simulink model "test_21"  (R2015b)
settings: Solver=FixedStepDiscrete  StartTime=0.0  StopTime=400.0  RelTol=1e-3
undefined symbols (not defined in the file or in its folder): fir1
libraries: simulink x1, dspstat3 x1

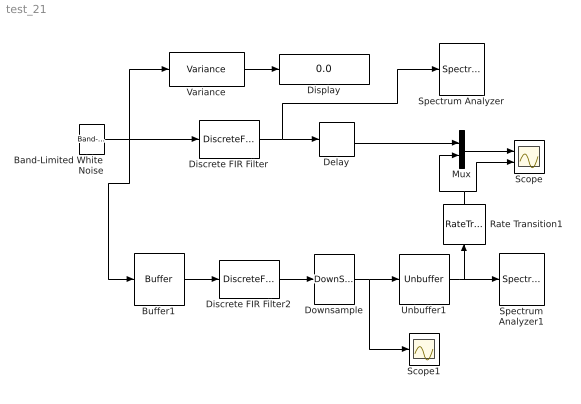
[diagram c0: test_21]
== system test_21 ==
  Band-Limited White Noise : simulink/Sources/Band-Limited White Noise  Cov=[0.01]  Ts=0.01  seed=[23341]
  Buffer1 : Buffer  N=2048  TreatMby1Signals=One channel  OutputFrames=off
  Delay : Delay  DelayLength=9*2048+4
  Discrete FIR Filter : DiscreteFir  Coefficients=fir1(256, 0.2);
  Discrete FIR Filter2 : DiscreteFir  Coefficients=fir1(256, 0.2);  InputProcessing=Columns as channels (frame based)
  Display : Display
  Downsample : DownSample  N=4  RateOptions=Allow multirate processing
  Mux : Mux  Inputs=2
  Rate Transition1 : RateTransition
  Scope : Scope  NumInputPorts=2
  Scope1 : Scope
  Spectrum Analyzer : SpectrumAnalyzer
  Spectrum Analyzer1 : SpectrumAnalyzer
  Unbuffer1 : Unbuffer  SampleBasedProcessing=Same as frame based
  Variance : dspstat3/Variance  run=on  reset_popup=None  directionMode=Each column  dimension=1  roiEnable=off  roiType=Rectangles  roiPortion=Entire ROI  roiOutput=Individual statistics for each ROI  roiFlag=off  roundingMode=Floor  overflowMode=off
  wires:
  Band-Limited White Noise/1 -> Variance/1, Discrete FIR Filter/1, Buffer1/1
  Mux/1 -> Scope/1
  Variance/1 -> Display/1
  Buffer1/1 -> Discrete FIR Filter2/1
  Discrete FIR Filter2/1 -> Downsample/1
  Downsample/1 -> Scope1/1, Unbuffer1/1
  Discrete FIR Filter/1 -> Delay/1, Spectrum Analyzer/1
  Unbuffer1/1 -> Rate Transition1/1, Spectrum Analyzer1/1
  Delay/1 -> Mux/1
  Rate Transition1/1 -> Mux/2, Scope/2
